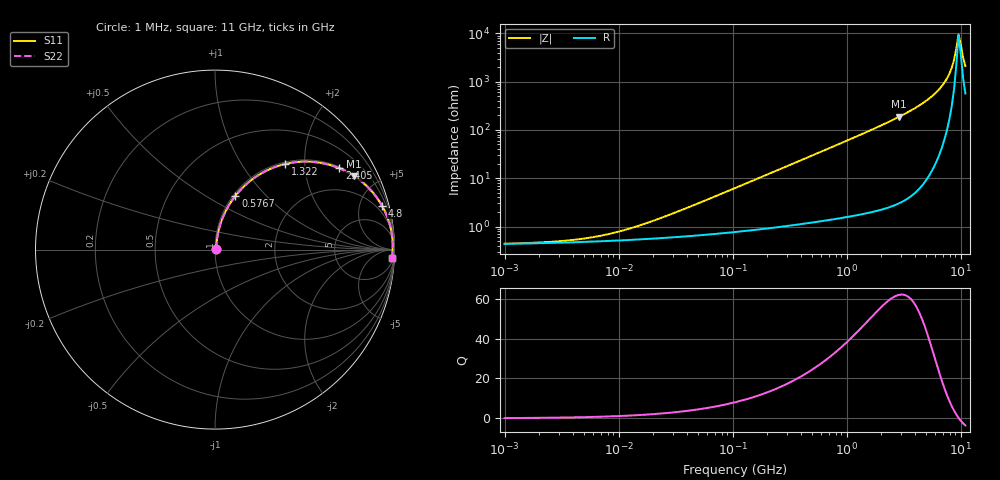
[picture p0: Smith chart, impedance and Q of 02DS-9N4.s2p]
# MHz S MA R 50
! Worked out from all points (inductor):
!   203 points, 1 MHz to 11 GHz, reference 50 ohm
!   read as one part in series: L = 9.4 nH near 31.66 MHz
!   highest Q = 61.9 at 2.892 GHz (marker M1), where L = 10.3 nH
!   self-resonance near 9.58 GHz
!   S11 on the Smith chart (normalised r, x): 1 MHz: 1.01, +0.00; 576.7 MHz: 1.03, +0.68; 1.322 GHz: 1.04, +1.59; 2.405 GHz: 1.05, +3.03; 4.8 GHz: 1.16, +7.54; 11 GHz: 12, -40
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1  0.004381 7.7  0.9957 -0.0  0.9957 -0.0  0.004381 7.7
4.78889  0.005534 30.4  0.9952 -0.2  0.9952 -0.2  0.005534 30.4
10.0079  0.007792 48.7  0.9949 -0.3  0.9949 -0.3  0.007792 48.7
22.9334  0.01462 66.3  0.9942 -0.8  0.9942 -0.8  0.01462 66.3
104.881  0.06183 79.4  0.9905 -3.5  0.9905 -3.5  0.06183 79.4
240.337  0.1396 78.1  0.9808 -8.0  0.9808 -8.0  0.1396 78.1
502.263  0.2822 71.3  0.9479 -16.4  0.9479 -16.4  0.2822 71.3
576.702  0.32 69.2  0.9356 -18.7  0.9356 -18.7  0.32 69.2
872.998  0.4561 61.2  0.877 -27.1  0.877 -27.1  0.4561 61.2
1321.53  0.616 50.7  0.7742 -38.0  0.7742 -38.0  0.616 50.7
1824.42  0.7384 41.3  0.6606 -47.6  0.6606 -47.6  0.7384 41.3
2405.28  0.8282 33.1  0.5467 -55.9  0.5467 -55.9  0.8282 33.1
2891.96  0.8767 27.8  0.4671 -61.2  0.4671 -61.2  0.8767 27.8
4800.3  0.9615 14.8  0.2551 -74.0  0.2551 -74.0  0.9615 14.8
6328.63  0.9827 8.6  0.1498 -79.1  0.1498 -79.1  0.9827 8.6
7609.17  0.9893 4.8  0.0835 -80.2  0.0835 -80.2  0.9893 4.8
8343.56  0.9905 2.9  0.05137 -77.9  0.05137 -77.9  0.9905 2.9
8736.92  0.9906 2.0  0.03571 -73.8  0.03571 -73.8  0.9906 2.0
9148.82  0.9904 1.1  0.02083 -62.1  0.02083 -62.1  0.9904 1.1
9580.14  0.9899 0.1  0.01045 -14.4  0.01045 -14.4  0.9899 0.1
10504.8  0.9878 -1.7  0.03152 66.4  0.03152 66.4  0.9878 -1.7
11000  0.9862 -2.6  0.04692 71.7  0.04692 71.7  0.9862 -2.6
